|Texas Instruments Incorporated
|Single-Channel, 16-Bit Programmable Current Output and Voltage Output
|   DIGITAL-TO-ANALOG CONVERTER for 4-mA to 20-mA Current Loop Applications
| Marketing part#   Digital Voltage   #bits  Output   Package   #pins
|   Range   type
|DAC8750IRHAR   2.7V to 5.5V   16   Current   QFN   40
|DAC8750IRHAT   2.7V to 5.5V   16   Current   QFN   40
|DAC8750IPWP   2.7V to 5.5V   16   Current   TSSOP   24
|DAC8750IPWPR   2.7V to 5.5V   16   Current   TSSOP   24
|DAC8760IRHAR   2.7V to 5.5V   16   Voltage/Current QFN   40
|DAC8760IRHAT   2.7V to 5.5V   16   Voltage/Current QFN   40
|DAC8760IPWP   2.7V to 5.5V   16   Voltage/Current TSSOP   24
|DAC8760IPWPR   2.7V to 5.5V   16   Voltage/Current TSSOP   24
[IBIS Ver]   4.0
[File name]   dac8750_60.ibs
|SimDE V3.0 201101 build 453
[File Rev]   1.0
[Date]   07/09/2011
[Source]   Texas Instruments Incorporated.
   Analog-eLab, HPA
   12500 TI Blvd
   Dallas, TX -75243
   For Support e-mail: elab_ibis@list.ti.com
[Notes]   Revision History:
   1.0: 07/09/2011
   - Initial version of the model
   - Initial Model generated from simulations in TISPICED
   - Model names with a trailing _3 contains the model for
   3V (2.7V and 3.3V) operation.
   _ Model names with trailing _5 contains
   the model for 5V (4.5V and 5.5V) operation.
   - Model not matched to measurements
   - C_comp although listed in numerical order of value are
   obtained from varying PVT conditions. For PVT conditions
   for each specific value refer the buffer description under
   respective [Model]. IBIS model user is responsible for using
   appropriate C_comp to simulate for Signal Integrity.
[Disclaimer]
  This model is designed as an aid for customers of Texas Instruments.
  TI and its licensors and suppliers make no warranties, either expressed
  or implied, with respect to this model, including the warranties of
  merchantability or fitness for a particular purpose.  The model is
  provided solely on an "as is" basis.  The entire risk as to its quality
  and performance is with the customer.
[Copyright] (C) Copyright 2011 Texas Instruments Incorporated.
   All rights reserved.
|   DAC8750 and DAC8760
[Component]   dac8750rta
[Manufacturer] TI
[Package]   | 40 QFN - RTA package
| variable   typ   min   max
R_pkg  0.05142   0.00124   0.13484
L_pkg  1.11207nH 0.26560nH 2.51164nH
C_pkg  0.28906pF 0.13725pF 0.42873pF
|-------------------------PIN------------------------------------------------
[Pin] signal_name  model_name  R_pin  L_pin C_pin
1   NC   NC   0.00145  0.35323nH  0.26040pF
2   _ALARM   DOU_OD   0.08187  1.56180nH  0.38353pF
3   GND   GND   0.08178  1.54004nH  0.37467pF
4   GND   GND   0.07887  1.46891nH  0.25273pF
5   CLR   DIN   0.08120  1.49897nH  0.34859pF
6   LATCH   DIN   0.08359  1.54178nH  0.24500pF
7   SCLK   DIN   0.08353  1.55247nH  0.35821pF
8   DIN   DIN   0.08262  1.55497nH  0.26546pF
9   SDO   DOU   0.08081  1.54275nH  0.37245pF
10  NC   NC   0.00146  0.35627nH  0.14514pF
11  NC   NC   0.00147  0.35836nH  0.36671pF
12  GND   GND   0.03145  0.90772nH  0.28149pF
13  GND   GND   0.03184  0.90068nH  0.37809pF
14  GND   GND   0.05891  1.11857nH  0.23117pF
15  GND   GND   0.05809  1.09071nH  0.32570pF
16  ISET-R   TERM   0.06132  1.14399nH  0.22365pF
17  REFOUT   TERM   0.03279  0.86949nH  0.38020pF
18  REFIN   TERM   0.07835  1.47353nH  0.25574pF
19  NC   NC   0.00146  0.32457nH  0.18960pF
20  NC   NC   0.00146  0.35532nH  0.13725pF
21  NC   NC   0.00142  0.34688nH  0.37618pF
22  NC   NC   0.00142  0.31572nH  0.20386pF
23  DVDD-EN   DVDD_EN   0.12949  2.39813nH  0.41260pF
24  HART_IN   TERM   0.13484  2.47926nH  0.30494pF
25  R3_SENSE  TERM   0.13385  2.45031nH  0.40205pF
26  I_OUT   TERM   0.13187  2.41363nH  0.29765pF
27  BOOST   TERM   0.13130  2.41361nH  0.41308pF
28  CAP1   TERM   0.13241  2.45224nH  0.32317pF
29  CAP2   TERM   0.13452  2.51164nH  0.42873pF
30  NC   NC   0.00144  0.35022nH  0.14686pF
31  NC   NC   0.00143  0.34950nH  0.36969pF
32  NC   NC   0.00143  0.31844nH  0.20234pF
33  NC   NC   0.00137  0.29721nH  0.29340pF
34  NC   NC   0.00129  0.27741nH  0.17831pF
35  NC   NC   0.00124  0.26560nH  0.27320pF
36  AVDD   POWER   0.03087  0.81872nH  0.25022pF
37  NC   NC   0.02980  0.80889nH  0.36549pF
38  NC   NC   0.00137  0.29738nH  0.18561pF
39  DVDD   POWER   0.05965  1.16548nH  0.24599pF
40  NC   NC   0.00145  0.35274nH  0.14084pF
[Component]   dac8760rta
[Manufacturer] TI
[Package]   | 40 QFN - RTA package
| variable   typ   min   max
R_pkg  0.05142   0.00124   0.13484
L_pkg  1.11207nH 0.26560nH 2.51164nH
C_pkg  0.28906pF 0.13725pF 0.42873pF
|-------------------------PIN------------------------------------------------
[Pin] signal_name  model_name  R_pin  L_pin C_pin
1   NC   NC   0.00145  0.35323nH  0.26040pF
2   _ALARM   DOU_OD   0.08187  1.56180nH  0.38353pF
3   GND   GND   0.08178  1.54004nH  0.37467pF
4   GND   GND   0.07887  1.46891nH  0.25273pF
5   CLR   DIN   0.08120  1.49897nH  0.34859pF
6   LATCH   DIN   0.08359  1.54178nH  0.24500pF
7   SCLK   DIN   0.08353  1.55247nH  0.35821pF
8   DIN   DIN   0.08262  1.55497nH  0.26546pF
9   SDO   DOU   0.08081  1.54275nH  0.37245pF
10  NC   NC   0.00146  0.35627nH  0.14514pF
11  NC   NC   0.00147  0.35836nH  0.36671pF
12  GND   GND   0.03145  0.90772nH  0.28149pF
13  GND   GND   0.03184  0.90068nH  0.37809pF
14  GND   GND   0.05891  1.11857nH  0.23117pF
15  GND   GND   0.05809  1.09071nH  0.32570pF
16  ISET-R   TERM   0.06132  1.14399nH  0.22365pF
17  REFOUT   TERM   0.03279  0.86949nH  0.38020pF
18  REFIN   TERM   0.07835  1.47353nH  0.25574pF
19  NC   NC   0.00146  0.32457nH  0.18960pF
20  NC   NC   0.00146  0.35532nH  0.13725pF
21  NC   NC   0.00142  0.34688nH  0.37618pF
22  NC   NC   0.00142  0.31572nH  0.20386pF
23  DVDD-EN   DVDD_EN   0.12949  2.39813nH  0.41260pF
24  HART_IN   TERM   0.13484  2.47926nH  0.30494pF
25  R3_SENSE  TERM   0.13385  2.45031nH  0.40205pF
26  I_OUT   TERM   0.13187  2.41363nH  0.29765pF
27  BOOST   TERM   0.13130  2.41361nH  0.41308pF
28  CAP1   TERM   0.13241  2.45224nH  0.32317pF
29  CAP2   TERM   0.13452  2.51164nH  0.42873pF
30  NC   NC   0.00144  0.35022nH  0.14686pF
31  NC   NC   0.00143  0.34950nH  0.36969pF
32  NC   NC   0.00143  0.31844nH  0.20234pF
33  NC   NC   0.00137  0.29721nH  0.29340pF
34  NC   NC   0.00129  0.27741nH  0.17831pF
35  NC   NC   0.00124  0.26560nH  0.27320pF
36  AVDD   POWER   0.03087  0.81872nH  0.25022pF
37  NC   NC   0.02980  0.80889nH  0.36549pF
38  NC   NC   0.00137  0.29738nH  0.18561pF
39  DVDD   POWER   0.05965  1.16548nH  0.24599pF
40  NC   NC   0.00145  0.35274nH  0.14084pF
[Component]   dac8750pwp
[Manufacturer] TI
[Package]   | 24 TSSOP - PW package
| variable   typ   min   max
R_pkg  0.0634   0.0054   0.0804
L_pkg  2.0264nH 1.1423nH 2.8935nH
C_pkg  0.4221pF 0.3492pF 0.5184pF
|-------------------------PIN------------------------------------------------
[Pin] signal_name  model_name  R_pin  L_pin C_pin
1   GND   GND   0.04286  2.54189nH  0.54529pF
2   DVDD   POWER   0.07925  2.23494nH  0.42189pF
3   _ALARM   DOU_OD   0.06478  1.98369nH  0.41692pF
4   GND   GND   0.06069  1.91629nH  0.41228pF
5   GND   GND   0.05664  1.83629nH  0.40146pF
6   CLR   DIN   0.06084  1.90430nH  0.40683pF
7   LATCH   DIN   0.06835  2.03635nH  0.41418pF
8   SCLK   DIN   0.07218  2.11012nH  0.41695pF
9   DIN   DIN   0.07309  2.13727nH  0.42447pF
10  SDO   DOU   0.07312  2.13511nH  0.42436pF
11  GND   GND   0.04353  1.90666nH  0.46184pF
12  GND   GND   0.04419  2.59266nH  0.54946pF
13  ISET-R   TERM   0.07895  2.89353nH  0.51839pF
14  REFOUT   TERM   0.04544  1.94488nH  0.47697pF
15  REFIN   TERM   0.05909  1.88831nH  0.41128pF
16  DVDD-EN   DVDD_EN   0.06070  1.91784nH  0.41145pF
17  HART_IN   TERM   0.07536  2.16535nH  0.41926pF
18  R3_SENSE  TERM   0.06902  2.04761nH  0.41552pF
19  I_OUT   TERM   0.06105  1.90687nH  0.40783pF
20  BOOST   TERM   0.06145  1.91754nH  0.40800pF
21  CAP1   TERM   0.06912  2.06104nH  0.42324pF
22  CAP2   TERM   0.08039  2.25741nH  0.43169pF
23  NC   NC   0.00540  1.14225nH  0.34915pF
24  AVDD   POWER   0.05089  2.76921nH  0.56304pF
[Component]   dac8760pwp
[Manufacturer] TI
[Package]   | 24 TSSOP - PW package
| variable   typ   min   max
R_pkg  0.0634   0.0054   0.0804
L_pkg  2.0264nH 1.1423nH 2.8935nH
C_pkg  0.4221pF 0.3492pF 0.5184pF
|-------------------------PIN------------------------------------------------
[Pin] signal_name  model_name  R_pin  L_pin C_pin
1   GND   GND   0.04286  2.54189nH  0.54529pF
2   DVDD   POWER   0.07925  2.23494nH  0.42189pF
3   _ALARM   DOU_OD   0.06478  1.98369nH  0.41692pF
4   GND   GND   0.06069  1.91629nH  0.41228pF
5   GND   GND   0.05664  1.83629nH  0.40146pF
6   CLR   DIN   0.06084  1.90430nH  0.40683pF
7   LATCH   DIN   0.06835  2.03635nH  0.41418pF
8   SCLK   DIN   0.07218  2.11012nH  0.41695pF
9   DIN   DIN   0.07309  2.13727nH  0.42447pF
10  SDO   DOU   0.07312  2.13511nH  0.42436pF
11  GND   GND   0.04353  1.90666nH  0.46184pF
12  GND   GND   0.04419  2.59266nH  0.54946pF
13  ISET-R   TERM   0.07895  2.89353nH  0.51839pF
14  REFOUT   TERM   0.04544  1.94488nH  0.47697pF
15  REFIN   TERM   0.05909  1.88831nH  0.41128pF
16  DVDD-EN   DVDD_EN   0.06070  1.91784nH  0.41145pF
17  HART_IN   TERM   0.07536  2.16535nH  0.41926pF
18  R3_SENSE  TERM   0.06902  2.04761nH  0.41552pF
19  I_OUT   TERM   0.06105  1.90687nH  0.40783pF
20  BOOST   TERM   0.06145  1.91754nH  0.40800pF
21  CAP1   TERM   0.06912  2.06104nH  0.42324pF
22  CAP2   TERM   0.08039  2.25741nH  0.43169pF
23  NC   NC   0.00540  1.14225nH  0.34915pF
24  AVDD   POWER   0.05089  2.76921nH  0.56304pF
|   Model Selectors
[Model Selector]  DIN
DIN_3   3V digital input
DIN_5   5V digital input
|NOTES   Model DIN split into two Models DIN_3 and DIN_5
|   to accommodate the voltage range of 2.7V - 5.5V
|   DIN_3 operates in voltage range of 2.7 - 3 - 3.3
|   DIN_5 operates in voltage range of 4.5 - 5 - 5.5
|   The max pin frequency for Model DIN is 31MHz. Also the
|   voltage range and frequency is referenced with datasheet.
[Model Selector]  DOU
DOU_3  3V 3-state digital output
DOU_5  5V 3-state digital output
|NOTES   Model DOU split into two Models DOU_3 and DOU_5
|   to accommodate the voltage range of 2.7V - 5.5V
|   DOU_3 operates in voltage range of 2.7 - 3 - 3.3
|   DOU_5 operates in voltage range of 4.5 - 5 - 5.5
|   The max pin frequency for Model DOU is 31MHz. Also the
|   voltage range and frequency is referenced with datasheet.
[Model Selector]  DVDD_EN
DVDD_EN_3  3V digital input
DVDD_EN_5  5V digital input
|NOTES   Model DVDD_EN split into two Models DVDD_EN_3 and DVDD_EN_5
|   to accommodate the voltage range of 2.7V - 5.5V
|   DVDD_EN_3 operates in voltage range of 2.7 - 3 - 3.3
|   DVDD_EN_5 operates in voltage range of 4.5 - 5 - 5.5
|   The max pin frequency for Model DVDD_EN is 31MHz. Also the
|   voltage range and frequency is referenced with datasheet.
[Model Selector]  DOU_OD
DOU_OD_3  3V opem drain digital output
DOU_OD_5  5V opem drain digital output
|NOTES   Model DOU_OD split into two Models DOU_OD_3 and DOU_OD_5
|   to accommodate the voltage range of 2.7V - 5.5V
|   DOU_OD_3 operates in voltage range of 2.7 - 3 - 3.3
|   DOU_OD_5 operates in voltage range of 4.5 - 5 - 5.5
|   The max pin frequency for Model DOU_OD is 31MHz. Also the
|   voltage range and frequency is referenced with datasheet.
[Model Selector]  TERM
TERM_3  3V termniator
TERM_5  5V termniator
|   TERM Models
[Model] TERM_3  |3V termniator
Model_type Terminator
C_comp   1e-20   1e-20   1e-20
| variable   typ   min   max
[Voltage Range]   3V   2.7V   3.3V
[POWER Clamp Reference]  3V   2.7V   3.3V
[GND Clamp Reference]   0.0V   0.0V   0.0V
|Operating Temperature   27   125   -40
|Junction Temperature
[Temperature Range]   36   134   -40
[Model] TERM_5  |5V terminator
Model_type Terminator
C_comp   1e-20   1e-20   1e-20
| variable   typ   min   max
[Voltage Range]   5V   4.5V   5.5V
[POWER Clamp Reference]  5V   4.5V   5.5V
[GND Clamp Reference]   0.0V   0.0V   0.0V
|Operating Temperature   27   125   -40
|Junction Temperature
[Temperature Range]   36   134   -40
| Models and submodels in the file (10): DIN_3 (Input), DIN_5 (Input), DOU_3 (3-state), DOU_5 (3-state), DVDD_EN_3 (Input), DVDD_EN_5 (Input), DOU_OD_3 (Open_drain), DOU_OD_5 (Open_drain), TERM_3 (Terminator), TERM_5 (Terminator)
